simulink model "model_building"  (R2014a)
settings: Solver=ode45  StartTime=0.0  StopTime=10.0  RelTol=1e-3

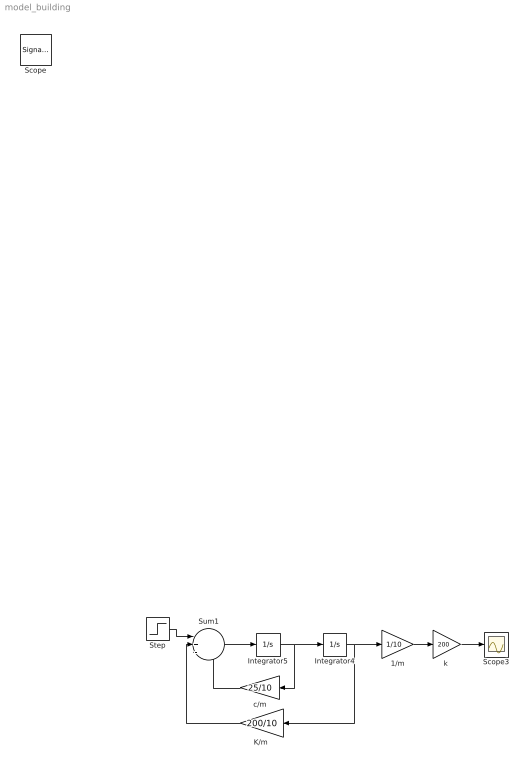
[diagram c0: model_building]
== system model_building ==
  1/m : Gain  Gain=1/10
  Integrator4 : Integrator
  Integrator5 : Integrator
  "K/m " : Gain  Gain=200/10
  Scope3 : Scope
  Step : Step  SampleTime=0
  Sum1 : Sum  Inputs=|+--
  c/m : Gain  Gain=25/10
  "k " : Gain  Gain=200
  Scope : SignalViewerScope  IOType=viewer  RefreshTime=0.035000
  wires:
  "k "/1 -> Scope3/1
  Integrator5/1 -> Integrator4/1, c/m/1
  c/m/1 -> Sum1/3
  Sum1/1 -> Integrator5/1
  "K/m "/1 -> Sum1/2
  Integrator4/1 -> 1/m/1, "K/m "/1
  1/m/1 -> "k "/1
  Step/1 -> Sum1/1
